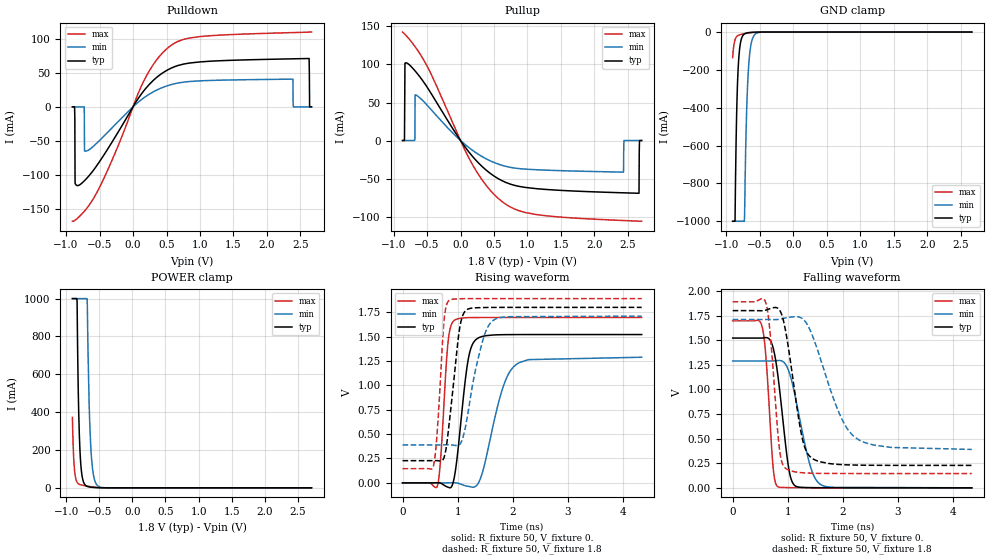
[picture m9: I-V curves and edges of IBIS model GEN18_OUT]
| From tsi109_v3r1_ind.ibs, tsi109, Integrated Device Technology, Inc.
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[Model]   GEN18_OUT
Model_type  Output
Polarity   Non-Inverting
Enable   Active-High
|   typ   min   max
|C_comp_off 3.714p 3.449p 3.979p
|C_comp_on 4.671p 4.263p 5.086p
C_comp 4.192p 3.856p 4.532p
Vinl  =   0.300v
Vinh  =   1.500v
Vmeas =   0.9000V
Cref  =   1.0pF
Rref  =   50.0000
Vref  =   0.0V
[Model Spec]
[Temperature Range]   25   125   -40
[Voltage Range] 1.8 1.71 1.89
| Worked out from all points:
|   slope of the pulldown table from 0 to 0.27 V, typ, clamps not added: 7.56 ohm
|   slope of the pullup table from 0 to 0.27 V, typ, clamps not added: 9.12 ohm
|   GND clamp passes 1 mA (typ) near -0.59 V on its own axis
|   POWER clamp passes 1 mA (typ) near -0.54 V on its own axis
|   rising waveform, R_fixture 50, V_fixture 0.: 20-80 % time 178ps typ, 338ps min, 109ps max; typ from 0 V to 1.52 V
|   rising waveform, R_fixture 50, V_fixture 1.8: 20-80 % time 179ps typ, 281ps min, 111ps max; typ from 0.228 V to 1.8 V
|   falling waveform, R_fixture 50, V_fixture 0.: 20-80 % time 187ps typ, 296ps min, 116ps max; typ from 1.52 V to 0 V
|   falling waveform, R_fixture 50, V_fixture 1.8: 20-80 % time 255ps typ, 510ps min, 145ps max; typ from 1.8 V to 0.228 V
[Pulldown]
-905.5mV  0A         0A         -168.3mA
-873mV    0A         0A         -167.3mA
-869.3mV  -15.33mA   0A         -167mA
-865.7mV  -112.5mA   0A         -166.8mA
-815.2mV  -115.6mA   0A         -162.6mA
-728.5mV  -109mA     0A         -153.7mA
-724.9mV  -108.6mA   -64.94mA   -153.3mA
-696mV    -105.6mA   -65mA      -149.9mA
531.9mV   55.13mA    31.64mA    87.73mA
2.63V     71.14mA    0A         109.9mA
2.637V    0A         0A         110mA
2.666V    0A         0A         110.1mA
[Pullup]
-866.2mV  0A         0A         142.6mA
-837.3mV  0A         0A         140.3mA
-830.1mV  101.7mA    0A         139.7mA
-801.2mV  101.8mA    0A         136.9mA
-685.7mV  92.24mA    0A         124.3mA
-674.8mV  91.13mA    60.07mA    122.9mA
621.7mV   -52.88mA   -32.62mA   -80.33mA
2.435V    -68.76mA   -41.53mA   -105.2mA
2.442V    -68.78mA   0A         -105.2mA
2.666V    -69.35mA   0A         -106mA
2.673V    0A         0A         -106.1mA
2.705V    0A         0A         -106.2mA
[GND Clamp]
-905.5mV  -1A        -1A        -135.4mA
-869.8mV  -997.8mA   -1A        -40.78mA
-846.1mV  -434.7mA   -1A        -24.25mA
-818.4mV  -161.8mA   -1A        -16.97mA
-786.7mV  -53.78mA   -1A        -13.18mA
-735.3mV  -11.55mA   -1A        -9.218mA
-727.3mV  -9.494mA   -973.7mA   -8.691mA
-699.6mV  -5.303mA   -454.7mA   -6.959mA
-671.9mV  -3.32mA    -208.8mA   -5.397mA
-632.3mV  -1.845mA   -67.93mA   -3.496mA
-565.1mV  -634.9uA   -10.08mA   -1.288mA
2.666V    0A         0A         0A
[Power Clamp]
-905.5mV  1A         1A         372.3mA
-880.8mV  1A         1A         126.4mA
-837.6mV  1A         1A         31.59mA
-816mV    494.2mA    1A         21.92mA
-791.4mV  197.7mA    1A         17.19mA
-757.4mV  58.87mA    1A         13.9mA
-701.9mV  11.65mA    1A         10.21mA
-683.4mV  7.9mA      1A         9.121mA
-652.6mV  4.758mA    440.2mA    7.418mA
-624.8mV  3.297mA    198.7mA    6.001mA
-520mV    740.6uA    9.847mA    1.874mA
2.705V    0A         0A         0A
[Ramp]
dV/dt_r .913/177.771p .773/338.311p 1.018/108.877p
dV/dt_f .943/254.559p .793/510.536p 1.047/145.208p
[Rising Waveform]
R_fixture = 50
V_fixture = 0.
0s        0V         0V         0V
630ps     1.026mV    -11.3uV    -38.16mV
700ps     -5.507mV   -139.2uV   311mV
820ps     -43.09mV   483.7uV    1.412V
940ps     57.21mV    823.1uV    1.667V
1.18ns    1.225V     -34.59mV   1.694V
1.35ns    1.477V     -23.74mV   1.696V
1.81ns    1.52V      956.8mV    1.696V
2.05ns    1.521V     1.208V     1.696V
4.34ns    1.521V     1.288V     1.696V
[Rising Waveform]
R_fixture = 50
V_fixture = 1.8
V_fixture_min = 1.71
V_fixture_max = 1.89
0s        227.8mV    389.2mV    145.4mV
560ps     228.5mV    389.2mV    171.1mV
630ps     227.7mV    389.2mV    528.7mV
760ps     273.7mV    389.9mV    1.701V
840ps     576.4mV    390.1mV    1.87V
1.04ns    1.597V     396.1mV    1.888V
1.17ns    1.777V     658.9mV    1.89V
1.45ns    1.798V     1.448V     1.89V
1.67ns    1.8V       1.675V     1.89V
4.34ns    1.8V       1.71V      1.89V
[Falling Waveform]
R_fixture = 50
V_fixture = 0.
0s        1.521V     1.289V     1.696V
540ps     1.522V     1.289V     1.625V
600ps     1.526V     1.289V     1.357V
740ps     1.411V     1.289V     174.2mV
820ps     1.145V     1.293V     10.89mV
1.02ns    188.8mV    1.183V     2.031mV
1.14ns    18.25mV    915.9mV    1.027mV
1.42ns    2.208mV    201.7mV    230.8uV
1.62ns    993.3uV    26.39mV    82.63uV
4.34ns    0V         13.39uV    0V
[Falling Waveform]
R_fixture = 50
V_fixture = 1.8
V_fixture_min = 1.71
V_fixture_max = 1.89
0s        1.8V       1.71V      1.89V
600ps     1.804V     1.71V      1.882V
680ps     1.82V      1.71V      1.573V
840ps     1.813V     1.712V     437.8mV
960ps     1.596V     1.725V     197.7mV
1.26ns    511.6mV    1.721V     153.4mV
1.44ns    300.7mV    1.556V     148.4mV
1.92ns    238mV      776.1mV    145.7mV
2.24ns    231.1mV    505.4mV    145.5mV
4.34ns    227.8mV    390.2mV    145.4mV
